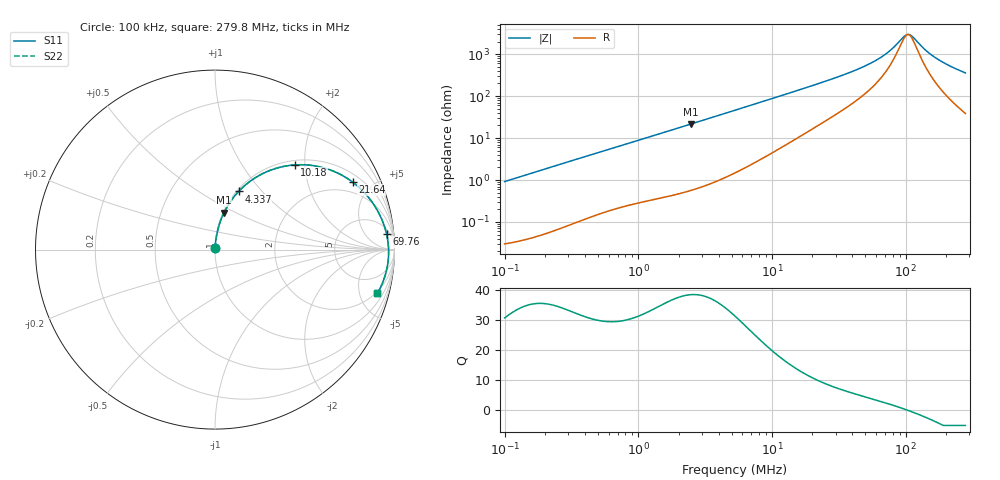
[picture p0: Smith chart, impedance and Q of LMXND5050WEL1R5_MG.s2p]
! LMXND5050WEL1R5_MG  S-PARAMETER MODEL  ( General Type )
! Model Generated by TAIYO YUDEN Corporation (https://www.yuden.co.jp/en/)
! Version 1.0
! TAIYO YUDEN Control No. 191023NI43SB-FBB
! Copyright(c) 2019 TAIYO YUDEN CO.,LTD. All Rights Reserved.
! Product Description (link to TY-COMPAS)
! https://ds.yuden.co.jp/TYCOMPAS/or/detail?pn=LMXND5050WEL1R5NMG&u=M
! Products Name : Inductors
! Characteristics :
!  Inductance : 1.5 uH , SRF(min) : 67 MHz , DC Resistance(max) : 0.0264 Ohm
!  Rated Current : Saturation :5200 mA , Temp Rise : 3600 mA (40 degC)
!  Case Size : 4.9 x 4.9 / 0.193 x 0.193 [mm/inch] , Thickness : 2.5 / 0.098 [mm/inch]
!  (Conditions: Temperature = 25 degC , DC Bias Current/Voltage = 0A / 0V)
! External Node Assignments :
!  1  o---GGG---o  2
! GND o---------o GND
! Frequency Range : 0.1MHz  -  279.750408MHz  [ 402 STEP ]
# MHz S RI R 50
! Freq[MHz].  S11 Real  S11 Imag  S21 Real  S21 Imag  S12 Real  S12 Imag  S22 Real  S22 Imag
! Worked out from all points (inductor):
!   401 points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, 100 kHz to 279.8 MHz, reference 50 ohm
!   read as one part in series: L = 1.46 uH near 104 kHz
!   highest Q = 38.3 at 2.489 MHz (marker M1), where L = 1.39 uH
!   self-resonance near 104 MHz
!   S11 on the Smith chart (normalised r, x): 100 kHz: 1.00, +0.02; 4.337 MHz: 1.02, +0.75; 10.18 MHz: 1.09, +1.78; 21.64 MHz: 1.38, +3.84; 69.76 MHz: 8, +18; 279.8 MHz: 1.77, -7.11
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0.1  0.000383 0.00916  0.9996 -0.00916  0.9996 -0.00916  0.000383 0.00916
0.377863  0.00225 0.0341  0.9977 -0.0341  0.9977 -0.0341  0.00225 0.0341
1.427803  0.0189 0.1224  0.9811 -0.1224  0.9811 -0.1224  0.0189 0.1224
2.488526  0.0498 0.205  0.9502 -0.205  0.9502 -0.205  0.0498 0.205
4.337266  0.1319 0.3241  0.8681 -0.3241  0.8681 -0.3241  0.1319 0.3241
5.289144  0.1827 0.3707  0.8173 -0.3707  0.8173 -0.3707  0.1827 0.3707
10.17991  0.4442 0.4719  0.5558 -0.4719  0.5558 -0.4719  0.4442 0.4719
13.98346  0.5945 0.4585  0.4055 -0.4585  0.4055 -0.4585  0.5945 0.4585
19.9857  0.7398 0.3949  0.2602 -0.3949  0.2602 -0.3949  0.7398 0.3949
21.63651  0.7664 0.3764  0.2336 -0.3764  0.2336 -0.3764  0.7664 0.3764
30.31621  0.8556 0.2906  0.1444 -0.2906  0.1444 -0.2906  0.8556 0.2906
44.19738  0.9171 0.195  0.0829 -0.195  0.0829 -0.195  0.9171 0.195
57.20271  0.9426 0.1336  0.0574 -0.1336  0.0574 -0.1336  0.9426 0.1336
69.75669  0.9556 0.0885  0.0444 -0.0885  0.0444 -0.0885  0.9556 0.0885
75.51853  0.9593 0.0708  0.0407 -0.0708  0.0407 -0.0708  0.9593 0.0708
97.74029  0.9666 0.0137  0.0334 -0.0137  0.0334 -0.0137  0.9666 0.0137
105.8136  0.9673 -0.00384  0.0327 0.00384  0.0327 0.00384  0.9673 -0.00384
112.3032  0.9674 -0.0171  0.0326 0.0171  0.0326 0.0171  0.9674 -0.0171
139.6942  0.9643 -0.0667  0.0357 0.0667  0.0357 0.0667  0.9643 -0.0667
167.0054  0.9572 -0.109  0.0428 0.109  0.0428 0.109  0.9572 -0.109
211.9014  0.9399 -0.1689  0.0601 0.1689  0.0601 0.1689  0.9399 -0.1689
279.7504  0.9048 -0.2442  0.0952 0.2442  0.0952 0.2442  0.9048 -0.2442
